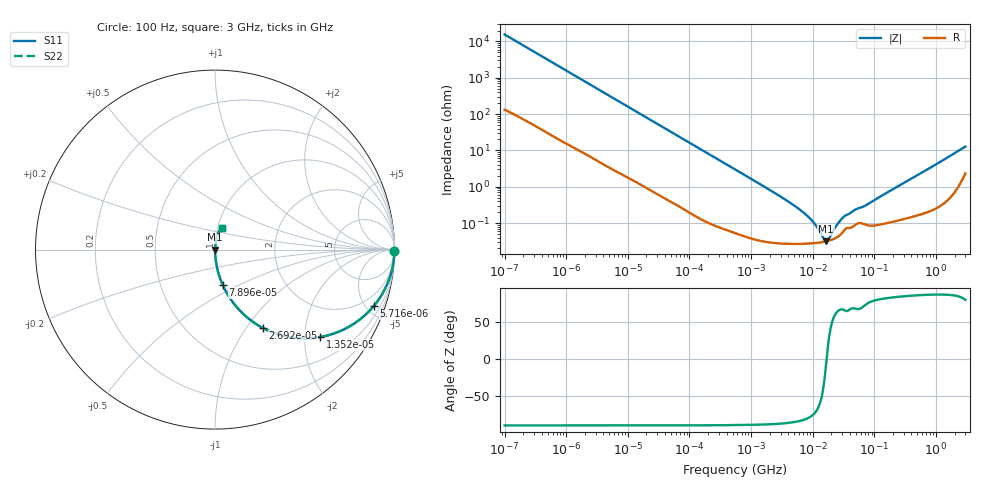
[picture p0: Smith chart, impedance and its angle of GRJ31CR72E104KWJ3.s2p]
!Murata Part Number: GRJ31CR72E104KWJ3
!These Parameters are Measured in Series Mode Connection
!Data Generated on Jun 19, 2026
!  o--ll--o
!Port1  Port2
!  o------o
!Operation Temp=25[degC], DC Bias Voltage=0[V]
!Freq. Start=100[Hz] Stop=3[GHz] 401[Steps]
# Hz S RI R 50
!Freq.(Hz) S11(Real) S11(Imag) S21(Real) S21(Imag) S12(Real) S12(Imag) S22(Real) S22(Imag)
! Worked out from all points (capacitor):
!   401 points, 100 Hz to 3 GHz, reference 50 ohm
!   read as one part in series: C = 102 nF near 109 Hz
!   lowest |Z| = 31.7 mohm at 16.42 MHz (marker M1)
!   series resonance near 16.8 MHz, so ESL is about 880 pH
!   S11 on the Smith chart (normalised r, x): 100 Hz: open; 5.716 kHz: 1.06, -5.59; 13.52 kHz: 1.03, -2.38; 26.92 kHz: 1.01, -1.20; 78.96 kHz: 1.00, -0.41; 3 GHz: 1.05, +0.25
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100  0.9999 -0.00642  9.57e-05 0.00642  9.57e-05 0.00642  0.9999 -0.00642
584  0.9983 -0.037  0.00173 0.037  0.00173 0.037  0.9983 -0.037
1788  0.9863 -0.1111  0.0137 0.1111  0.0137 0.1111  0.9863 -0.1111
5716  0.8839 -0.3151  0.1161 0.3151  0.1161 0.3151  0.8839 -0.3151
8791  0.766 -0.4179  0.234 0.4179  0.234 0.4179  0.766 -0.4179
13520  0.5846 -0.4871  0.4154 0.4871  0.4154 0.4871  0.5846 -0.4871
26919  0.2671 -0.4367  0.7329 0.4367  0.7329 0.4367  0.2671 -0.4367
31977  0.2064 -0.399  0.7936 0.399  0.7936 0.399  0.2064 -0.399
78956  0.043 -0.1969  0.957 0.1969  0.957 0.1969  0.043 -0.1969
186741  0.00867 -0.0868  0.9913 0.0868  0.9913 0.0868  0.00867 -0.0868
547723  0.00143 -0.03  0.9986 0.03  0.9986 0.03  0.00143 -0.03
4323298  0.00028 -0.00359  0.9997 0.00359  0.9997 0.00359  0.00028 -0.00359
6941223  0.000272 -0.00198  0.9997 0.00198  0.9997 0.00198  0.000272 -0.00198
9794414  0.000278 -0.00112  0.9997 0.00112  0.9997 0.00112  0.000278 -0.00112
1.506283e7  0.000304 -0.000217  0.9997 0.000217  0.9997 0.000217  0.000304 -0.000217
1.641694e7  0.000313 -4.54e-05  0.9997 4.54e-05  0.9997 4.54e-05  0.000313 -4.54e-05
1.789277e7  0.000325 0.000126  0.9997 -0.000126  0.9997 -0.000126  0.000325 0.000126
2.52476e7  0.000415 0.000843  0.9996 -0.000843  0.9996 -0.000843  0.000415 0.000843
3.268714e7  0.000645 0.0014  0.9994 -0.0014  0.9994 -0.0014  0.000645 0.0014
1.751444e8  0.00108 0.00742  0.9989 -0.00742  0.9989 -0.00742  0.00108 0.00742
9.384596e8  0.00385 0.0383  0.9961 -0.0383  0.9961 -0.0383  0.00385 0.0383
3e9  0.0371 0.1178  0.9629 -0.1178  0.9629 -0.1178  0.0371 0.1178
